// TwinCAT EventLogger功能记录中文内容
FUNCTION_BLOCK FB_EventInfo
VAR_INPUT
	sSourceName				:STRING;		// 日志产生源
	iID						:INT;			// 日志ID
	wsMsg					:WSTRING;		// 日志文本
END_VAR
VAR_OUTPUT
	bInited					:BOOL;			// 功能块初始化完成
END_VAR
VAR
	hr						:HRESULT;
	bNeedInit				:BOOL;
	sSrcNameTemp			:STRING;
	iIDTemp					:INT;
	fbSrcInfo				:FB_TcSourceInfo;
	fbTrig_Send				:R_TRIG;
	fbMsg					:FB_TcMessage;
END_VAR

// 检查是否完成初始化或需要重新初始化
bNeedInit := sSourceName <> sSrcNameTemp
				OR iID <> iIDTemp;
IF bNeedInit THEN
	bNeedInit := FALSE;
	fbSrcInfo.nId := iID;
	fbSrcInfo.sName := sSourceName;
	hr := fbMsg.CreateEx(tc_events.TcDemoEventClass.Info,fbSrcInfo);
	IF hr = 0 THEN
		bInited := TRUE;
		iIDTemp := iID;
		sSrcNameTemp := sSourceName;
	ELSE
		bInited := FALSE;
		RETURN;
	END_IF
END_IF

IF NOT bInited THEN
	RETURN;
END_IF

METHOD M_SendMsg : BOOL
VAR_INPUT
	
END_VAR
// 消息发送
IF bInited THEN
	fbMsg.ipArguments.Clear().AddWString(wsMsg);
	fbMsg.Send(0);
END_IF
END_METHOD

END_FUNCTION_BLOCK
